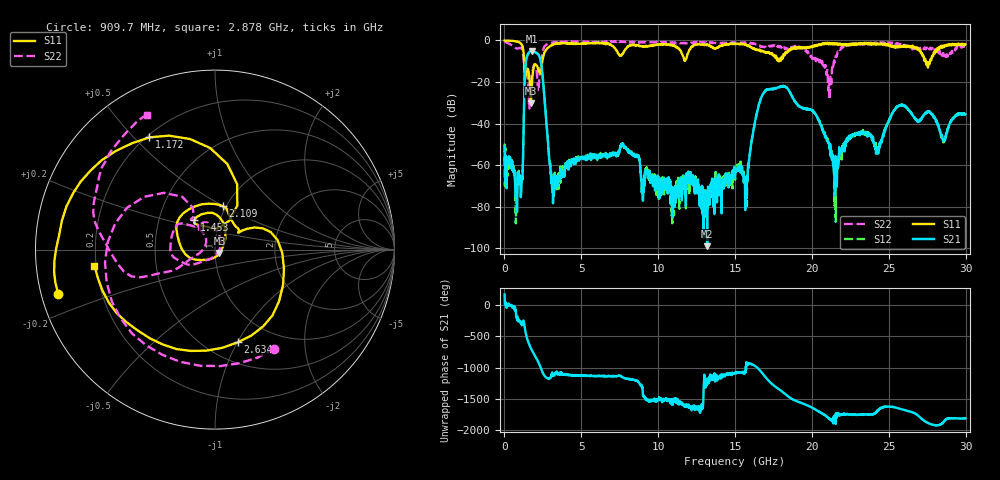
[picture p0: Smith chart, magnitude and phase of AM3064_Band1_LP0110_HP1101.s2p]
# Hz S DB R 50.0
!freq dBS11 angS11 dBS21 angS21 dBS12 angS12 dBS22 angS22
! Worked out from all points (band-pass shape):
!   1600 points, 10 MHz to 29.98 GHz, reference 50 ohm
!   highest |S21| = -5.14 dB at 1.791 GHz (marker M1); lowest = -98.9 dB at 13.19 GHz (marker M2)
!   |S21| within 3 dB of the highest: 1.452 GHz to 2.291 GHz (839.5 MHz wide, 44.9 % of centre)
!   lowest |S11| = -30.3 dB at 1.716 GHz (marker M3), VSWR 1.06, Z = 52.5 - j1.9 ohm
!   |S11| at or under -10 dB: 1.277 GHz to 2.46 GHz (1.184 GHz wide, 63.3 % of centre); 17.84566 GHz to 17.85704 GHz (11.37 MHz wide, 0.0637 % of centre); 27.4 GHz to 27.68 GHz (281.2 MHz wide, 1.02 % of centre)
!   |S22| runs from -32.7 to -0.4 dB; largest |S21 - S12| = 0.0092
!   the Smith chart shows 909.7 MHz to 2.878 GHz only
!   S11 on the Smith chart (normalised r, x): 909.7 MHz: 0.05, -0.14; 1.172 GHz: 0.21, +0.55; 1.453 GHz: 0.75, +0.26; 2.109 GHz: 0.97, +0.50; 2.634 GHz: 0.70, -1.00; 2.878 GHz: 0.19, -0.07
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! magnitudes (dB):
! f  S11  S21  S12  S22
! 10 MHz  -0.1  -51.0  -49.6  -0.4
! 909.7 MHz  -0.8  -66.6  -69.2  -3.8
! 1.172 GHz  -2.8  -66.8  -66.9  -4.8
! 1.453 GHz  -14.0  -8.1  -8.0  -15.8
! 1.716 GHz  -30.3  -5.2  -5.2  -20.9
! 1.791 GHz  -20.5  -5.1  -5.2  -16.1
! 2.109 GHz  -12.2  -6.1  -6.1  -16.1
! 2.634 GHz  -5.5  -30.7  -30.6  -2.7
! 2.878 GHz  -3.4  -52.6  -53.7  -1.5
! 3.196 GHz  -1.9  -65.5  -67.3  -1.2
! 5.015 GHz  -1.4  -56.2  -57.6  -0.7
! 7.714 GHz  -6.3  -49.5  -50.5  -0.8
! 10 GHz  -2.0  -66.9  -65.7  -1.0
! 13.19 GHz  -2.1  -98.9  -74.9  -1.1
! 15 GHz  -1.7  -63.4  -67.0  -1.4
! 15.74 GHz  -2.1  -75.6  -75.2  -1.1
! 17.01 GHz  -6.1  -23.9  -23.8  -3.4
! 19.99 GHz  -3.3  -33.6  -33.5  -8.3
! 21.13 GHz  -1.3  -51.6  -49.4  -21.3
! 21.57 GHz  -2.0  -67.2  -60.9  -7.4
! 25 GHz  -2.0  -38.6  -38.6  -1.3
! 29.98 GHz  -1.8  -35.6  -35.4  -3.0
